(* Logix 5000 AddOnInstructionDefinition export; software revision 16.04 *)

ADD_ON_INSTRUCTION AMCI_ANG1E_Run_Dwell_Move   (* revision 1.1, vendor AMCI, ExecuteEnableInFalse *)
// Revision note:
// Version 1.1 added the slot_axis number and the input parameters can now be tags or discrete values.
VAR_INPUT
   Axis_Status_Bits : INT; {required}
   slot_axis_number : INT; {required}
   Assembed_Move_Dwell_Time : INT; {required}
   Type_0_for_standard_1_for_indexed : BOOL;
END_VAR
VAR_IN_OUT
   AMCI_ANG1E_output_data : INT[10]; {required}
END_VAR
VAR_OUTPUT
   EN : BOOL; {visible}
   ER : BOOL; {visible}
END_VAR
VAR
   command_data_block : INT[10];
        [0]   // Command Bits MSW
        [1]   // Command Bits LSW
        [2]   // Upper Target Position
        [3]   // Lower Target Position
        [4]   // Upper Programmed Speed
        [5]   // Lower Programmed Speed
   index : INT;
END_VAR

ROUTINE EnableInFalse   (* ladder *)
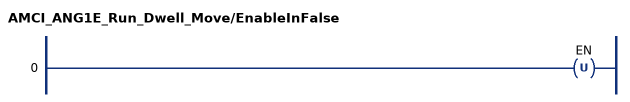
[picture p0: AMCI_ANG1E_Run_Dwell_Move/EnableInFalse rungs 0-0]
   0: OTU(EN);
END_ROUTINE

ROUTINE Logic   (* ladder *)
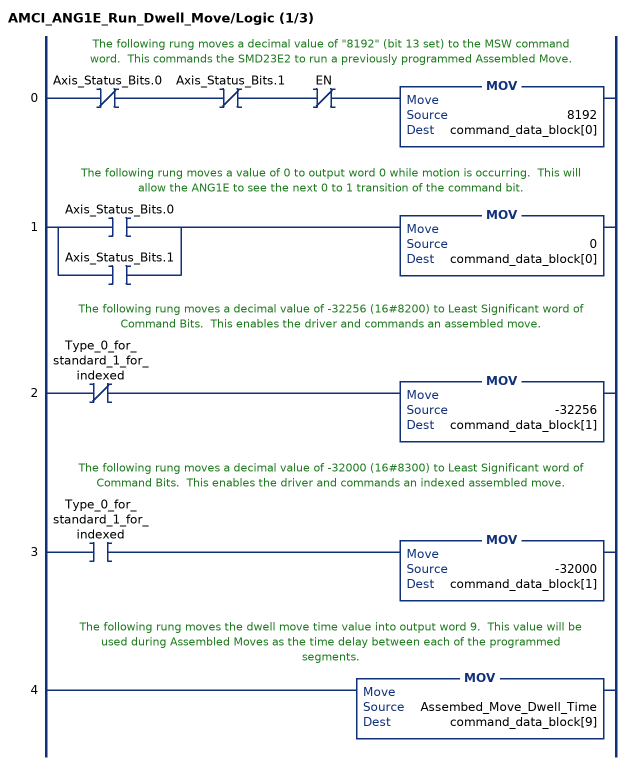
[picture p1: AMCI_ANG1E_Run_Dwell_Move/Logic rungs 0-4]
   // The following rung moves a decimal value of "8192" (bit 13 set) to the MSW command word.  This commands the SMD23E2 to run a previously programmed Assembled Move.
   0: XIO(Axis_Status_Bits.0)XIO(Axis_Status_Bits.1)XIO(EN)MOV(8192,command_data_block[0]);
   // The following rung moves a value of 0 to output word 0 while motion is occurring.  This will allow the ANG1E to see the next 0 to 1 transition of the command bit.
   1: [XIC(Axis_Status_Bits.0) ,XIC(Axis_Status_Bits.1) ]MOV(0,command_data_block[0]);
   // The following rung moves a decimal value of -32256 (16#8200) to Least Significant word of Command Bits.  This enables the driver and commands an assembled move.
   2: XIO(Type_0_for_standard_1_for_indexed)MOV(-32256,command_data_block[1]);
   // The following rung moves a decimal value of -32000 (16#8300) to Least Significant word of Command Bits.  This enables the driver and commands an indexed assembled move.
   3: XIC(Type_0_for_standard_1_for_indexed)MOV(-32000,command_data_block[1]);
   // The following rung moves the dwell move time value into output word 9.  This value will be used during Assembled Moves as the time delay between each of the programmed segments.
   4: MOV(Assembed_Move_Dwell_Time,command_data_block[9]);
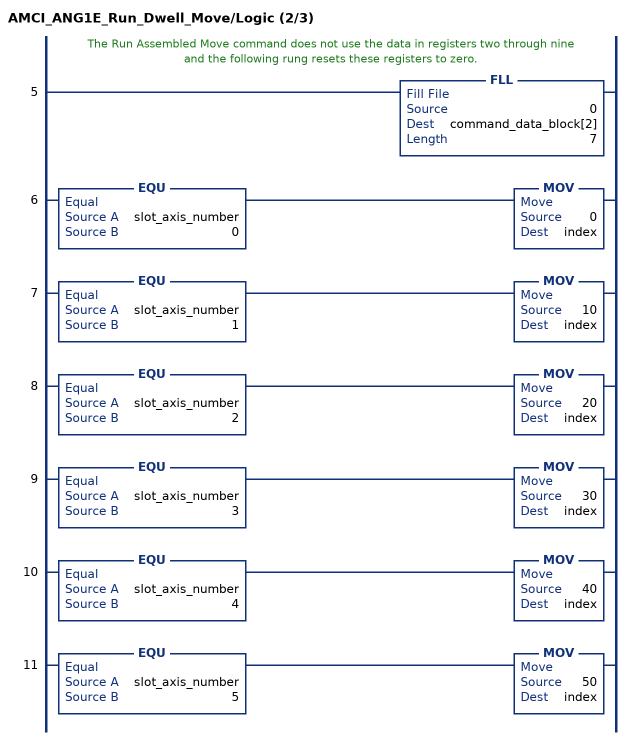
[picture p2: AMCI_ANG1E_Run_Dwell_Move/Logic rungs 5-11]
   // The Run Assembled Move command does not use the data in registers two through nine and the following rung resets these registers to zero.
   5: FLL(0,command_data_block[2],7);
   6: EQU(slot_axis_number,0)MOV(0,index);
   7: EQU(slot_axis_number,1)MOV(10,index);
   8: EQU(slot_axis_number,2)MOV(20,index);
   9: EQU(slot_axis_number,3)MOV(30,index);
   10: EQU(slot_axis_number,4)MOV(40,index);
   11: EQU(slot_axis_number,5)MOV(50,index);
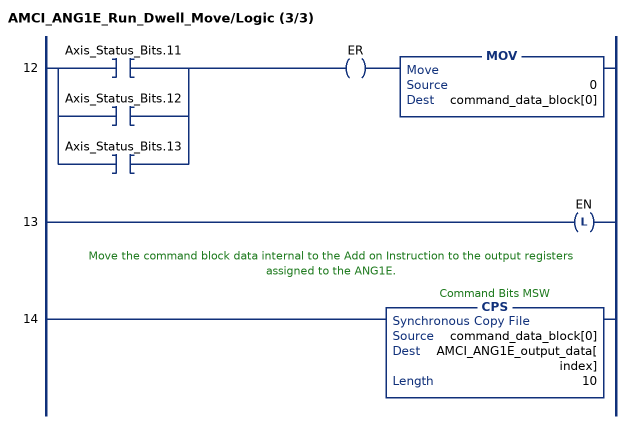
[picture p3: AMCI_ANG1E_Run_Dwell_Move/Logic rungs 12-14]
   12: [XIC(Axis_Status_Bits.11) ,XIC(Axis_Status_Bits.12) ,XIC(Axis_Status_Bits.13) ]OTE(ER)MOV(0,command_data_block[0]);
   13: OTL(EN);
   // Move the command block data internal to the Add on Instruction to the output registers assigned to the ANG1E.
   14: CPS(command_data_block[0],AMCI_ANG1E_output_data[index],10);
END_ROUTINE
END_ADD_ON_INSTRUCTION
